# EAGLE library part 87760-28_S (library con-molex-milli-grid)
HEADER
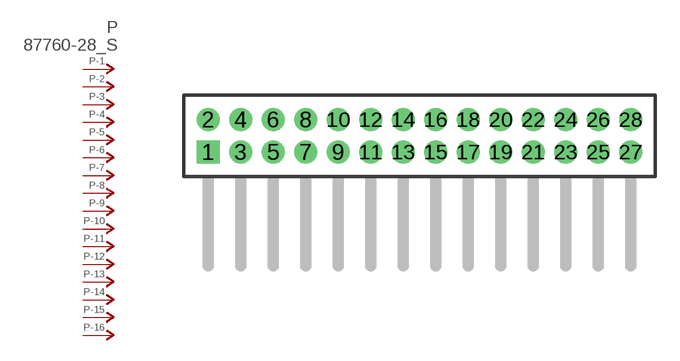
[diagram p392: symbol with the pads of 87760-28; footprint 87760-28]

Designator prefix P; gates -1=P-NV -2=P-N -3=P-N -4=P-N -5=P-N -6=P-N -7=P-N -8=P-N -9=P-N -10=P-N -11=P-N -12=P-N -13=P-N -14=P-N -15=P-N -16=P-N -17=P-N -18=P-N -19=P-N -20=P-N -21=P-N -22=P-N -23=P-N -24=P-N -25=P-N -26=P-N -27=P-N -28=P-N

## 87760-28_S  [87760-28]
1  -1:P  pas
2  -2:P  pas
3  -3:P  pas
4  -4:P  pas
5  -5:P  pas
6  -6:P  pas
7  -7:P  pas
8  -8:P  pas
9  -9:P  pas
10  -10:P  pas
11  -11:P  pas
12  -12:P  pas
13  -13:P  pas
14  -14:P  pas
15  -15:P  pas
16  -16:P  pas
17  -17:P  pas
18  -18:P  pas
19  -19:P  pas
20  -20:P  pas
21  -21:P  pas
22  -22:P  pas
23  -23:P  pas
24  -24:P  pas
25  -25:P  pas
26  -26:P  pas
27  -27:P  pas
28  -28:P  pas

## Footprint 87760-28 (pad centres in mm)
HEADER Dual Row, Right Angle
drill 0.914 square: 1 -13,-1
drill 0.914: 2 -13,1; 3 -11,-1; 4 -11,1; 5 -9,-1; 6 -9,1; 7 -7,-1; 8 -7,1; 9 -5,-1; 10 -5,1; 11 -3,-1; 12 -3,1; 13 -1,-1; 14 -1,1; 15 1,-1; 16 1,1; 17 3,-1; 18 3,1; 19 5,-1; 20 5,1; 21 7,-1; 22 7,1; 23 9,-1; 24 9,1; 25 11,-1; 26 11,1; 27 13,-1; 28 13,1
